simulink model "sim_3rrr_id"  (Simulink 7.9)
settings: Solver=ode45  StartTime=0.0  StopTime=2  RelTol=1e-3  AbsTol=1e-3
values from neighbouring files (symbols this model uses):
  m = 1    [mechanical_system.m]
  s = Lv/norm(Lv)    [pkm1.m]
undefined symbols (not defined in the file or in its folder): deg, kg, mN, N, rad
libraries: mblibv1 x26

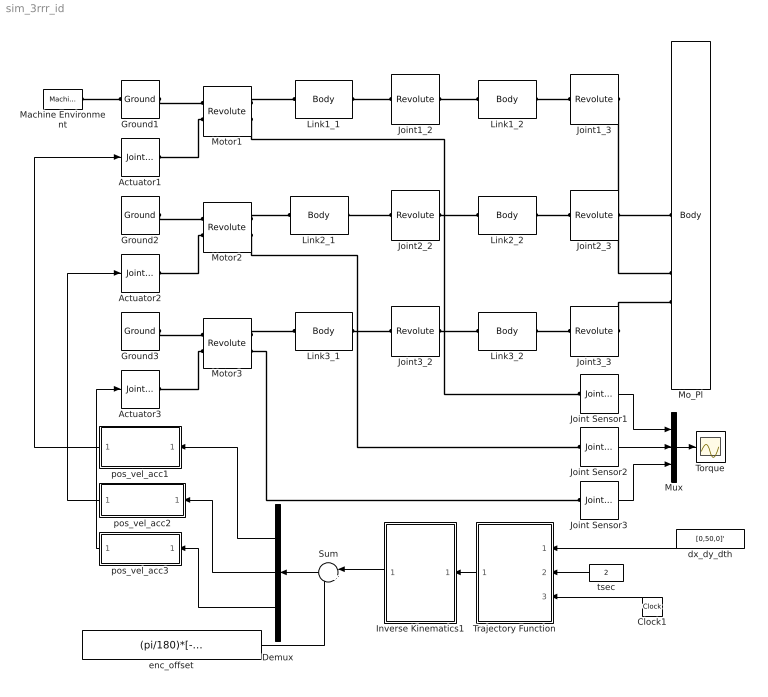
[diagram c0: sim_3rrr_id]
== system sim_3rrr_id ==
  Actuator1 : mblibv1/Sensors &  Actuators/Joint Actuator  UpdateFromCAD=off  PhysicalDomain=Mechanical  PortType=blob  ActuationStyle=Motion  AngleUnits=rad  ArcVelocityUnits=rad/s  ArcAccelerationUnits=rad/s^2  CoordPositionUnits=m  VelocityUnits=m/s  AccelerationUnits=m/s^2  ForceUnits=N  TorqueUnits=N*m  ActiveIO=on  Width=3  DialogClass=MechanicalActuatorBlock  Primitive=R1  ReferenceFrame=Absolute (World)
  Actuator2 : mblibv1/Sensors &  Actuators/Joint Actuator  UpdateFromCAD=off  PhysicalDomain=Mechanical  PortType=blob  ActuationStyle=Motion  AngleUnits=rad  ArcVelocityUnits=rad/s  ArcAccelerationUnits=rad/s^2  CoordPositionUnits=m  VelocityUnits=m/s  AccelerationUnits=m/s^2  ForceUnits=N  TorqueUnits=N*m  ActiveIO=on  Width=3  DialogClass=MechanicalActuatorBlock  Primitive=R1  ReferenceFrame=Absolute (World)
  Actuator3 : mblibv1/Sensors &  Actuators/Joint Actuator  UpdateFromCAD=off  PhysicalDomain=Mechanical  PortType=blob  ActuationStyle=Motion  AngleUnits=rad  ArcVelocityUnits=rad/s  ArcAccelerationUnits=rad/s^2  CoordPositionUnits=m  VelocityUnits=m/s  AccelerationUnits=m/s^2  ForceUnits=N  TorqueUnits=N*m  ActiveIO=on  Width=3  DialogClass=MechanicalActuatorBlock  Primitive=R1  ReferenceFrame=Absolute (World)
  Clock1 : Clock
  Demux : Demux  Outputs=3
  Ground1 : mblibv1/Bodies/Ground  UpdateFromCAD=off  LeftPortType=env  RightPortType=workingframe  PhysicalDomain=Mechanical  DialogClass=GroundBlock  CoordPosition=[0 0.15 0]  CoordPositionUnits=m  StateVectorMgrId=10  MachineId=[11 0]  ShowEnvPort=on
  Ground2 : mblibv1/Bodies/Ground  UpdateFromCAD=off  LeftPortType=env  RightPortType=workingframe  PhysicalDomain=Mechanical  DialogClass=GroundBlock  CoordPosition=[-0.1299 -0.075 0]  CoordPositionUnits=m  StateVectorMgrId=-1  MachineId=[0 0]  ShowEnvPort=off
  Ground3 : mblibv1/Bodies/Ground  UpdateFromCAD=off  LeftPortType=env  RightPortType=workingframe  PhysicalDomain=Mechanical  DialogClass=GroundBlock  CoordPosition=[0.129902 -0.074997 0]  CoordPositionUnits=m  StateVectorMgrId=-1  MachineId=[0 0]  ShowEnvPort=off
  Inverse Kinematics1 : MATLAB Function  TreatAsAtomicUnit=on
  Joint Sensor1 : mblibv1/Sensors &  Actuators/Joint Sensor  UpdateFromCAD=off  PhysicalDomain=Mechanical  PortType=blob  Muxed=on  Pose=off  Angle=off  AngleUnits=deg  ArcVelocity=off  ArcVelocityUnits=deg/s  ArcAcceleration=off  ArcAccelerationUnits=deg/s^2  CoordPosition=on  CoordPositionUnits=m  Velocity=off  VelocityUnits=m/s  Acceleration=off  AccelerationUnits=m/s^2  Quaternion=on  QuaternionDT=off  QuaternionDDT=off  QuaternionUnits=off  OutputVector=[1]  ActiveIO=on  Width=1  DialogClass=MechanicalSensorBlock  Primitive=R1  Force=off  ForceUnits=N  Torque=on  TorqueUnits=mN*m  ReferenceFrame=Absolute (World)  ReactionSensedSide=Base  ReactionReferenceFrame=Absolute (World)  ReactionForce=off  ReactionForceUnits=N  ReactionMoment=off  ReactionMomentUnits=N*m
  Joint Sensor2 : mblibv1/Sensors &  Actuators/Joint Sensor  UpdateFromCAD=off  PhysicalDomain=Mechanical  PortType=blob  Muxed=on  Pose=off  Angle=off  AngleUnits=deg  ArcVelocity=off  ArcVelocityUnits=deg/s  ArcAcceleration=off  ArcAccelerationUnits=deg/s^2  CoordPosition=on  CoordPositionUnits=m  Velocity=off  VelocityUnits=m/s  Acceleration=off  AccelerationUnits=m/s^2  Quaternion=on  QuaternionDT=off  QuaternionDDT=off  QuaternionUnits=off  OutputVector=[1]  ActiveIO=on  Width=1  DialogClass=MechanicalSensorBlock  Primitive=R1  Force=off  ForceUnits=N  Torque=on  TorqueUnits=mN*m  ReferenceFrame=Absolute (World)  ReactionSensedSide=Base  ReactionReferenceFrame=Absolute (World)  ReactionForce=off  ReactionForceUnits=N  ReactionMoment=off  ReactionMomentUnits=N*m
  Joint Sensor3 : mblibv1/Sensors &  Actuators/Joint Sensor  UpdateFromCAD=off  PhysicalDomain=Mechanical  PortType=blob  Muxed=on  Pose=off  Angle=off  AngleUnits=deg  ArcVelocity=off  ArcVelocityUnits=deg/s  ArcAcceleration=off  ArcAccelerationUnits=deg/s^2  CoordPosition=on  CoordPositionUnits=m  Velocity=off  VelocityUnits=m/s  Acceleration=off  AccelerationUnits=m/s^2  Quaternion=on  QuaternionDT=off  QuaternionDDT=off  QuaternionUnits=off  OutputVector=[1]  ActiveIO=on  Width=1  DialogClass=MechanicalSensorBlock  Primitive=R1  Force=off  ForceUnits=N  Torque=on  TorqueUnits=mN*m  ReferenceFrame=Absolute (World)  ReactionSensedSide=Base  ReactionReferenceFrame=Absolute (World)  ReactionForce=off  ReactionForceUnits=N  ReactionMoment=off  ReactionMomentUnits=N*m
  Joint1_2 : mblibv1/Joints/Revolute  LConnTagsString=__newl0  RConnTagsString=__newr0  UpdateFromCAD=off  NumSAPorts=0  CutJoint=off  MarkAsCut=off  Primitives=prismatic  PrimitiveProps=R1$World$[0 0 1]$revolute  DialogClass=JointBlock  R1Axis=[0 0 1]
  Joint1_3 : mblibv1/Joints/Revolute  LConnTagsString=__newl0  RConnTagsString=__newr0  UpdateFromCAD=off  NumSAPorts=0  CutJoint=off  MarkAsCut=off  Primitives=prismatic  PrimitiveProps=R1$World$[0 0 1]$revolute  DialogClass=JointBlock  R1Axis=[0 0 1]
  Joint2_2 : mblibv1/Joints/Revolute  LConnTagsString=__newl0  RConnTagsString=__newr0  UpdateFromCAD=off  NumSAPorts=0  CutJoint=off  MarkAsCut=off  Primitives=prismatic  PrimitiveProps=R1$World$[0 0 1]$revolute  DialogClass=JointBlock  R1Axis=[0 0 1]
  Joint2_3 : mblibv1/Joints/Revolute  LConnTagsString=__newl0  RConnTagsString=__newr0  UpdateFromCAD=off  NumSAPorts=0  CutJoint=off  MarkAsCut=off  Primitives=prismatic  PrimitiveProps=R1$World$[0 0 1]$revolute  DialogClass=JointBlock  R1Axis=[0 0 1]
  Joint3_2 : mblibv1/Joints/Revolute  LConnTagsString=__newl0  RConnTagsString=__newr0  UpdateFromCAD=off  NumSAPorts=0  CutJoint=off  MarkAsCut=off  Primitives=prismatic  PrimitiveProps=R1$World$[0 0 1]$revolute  DialogClass=JointBlock  R1Axis=[0 0 1]
  Joint3_3 : mblibv1/Joints/Revolute  LConnTagsString=__newl0  RConnTagsString=__newr0  UpdateFromCAD=off  NumSAPorts=0  CutJoint=off  MarkAsCut=off  Primitives=prismatic  PrimitiveProps=R1$World$[0 0 1]$revolute  DialogClass=JointBlock  R1Axis=[0 0 1]
  Link1_1 : mblibv1/Bodies/Body  LConnTagsString=CS1  RConnTagsString=CS2  UpdateFromCAD=off  DialogClass=MechanicalBodyBlock  Mass=0.053  MassUnits=kg  InertiaUnits=kg*m^2  Inertia=[0 0 0; 0 0 0; 0 0 0.000110621]  Shape=Cylinder  ShapeDims=[1 1]  ShapeUnits=m  ShapeUse=false  Density=1  DensityUnits=kg/m^3  DensityUse=false  GraphicsMode=MACHINE_DEFAULT  BodyColorSelMode=MACHINE_DEFAULT  BodyColor=[1 0 0]  AttachedToCS=CG  CG=Left$CG$[-0.043452 -0.030538 0]$CS1$CS1$m$[0 0 0]$Euler X-Y-Z$deg$WORLD$false$none  WorkingFrames=Left$CS1$[0 0.15 0]$World$World$m$[0 0 0]$Euler X-Y-Z$deg$WORLD$true$none#Right$CS2$[-0.081818 0.092497 0]$World$World$m$[0 0 0]$Euler X-Y-Z$deg$WORLD$true$none  CGPos=[-0.043452 -0.030538 0]  CGRot=[0 0 0]  CS0Pos=[]  CS0Rot=[]  CS1Pos=[0 0.15 0]  CS1Rot=[0 0 0]  CS2Pos=[-0.081818 0.092497 0]  CS2Rot=[0 0 0]  CS3Pos=[]  CS3Rot=[]  CS4Pos=[]  CS4Rot=[]  CS5Pos=[]  CS5Rot=[]  CS6Pos=[]  CS6Rot=[]  CS7Pos=[]  CS7Rot=[]  CS8Pos=[]  CS8Rot=[]  CS9Pos=[]  CS9Rot=[]  CS10Pos=[]  CS10Rot=[]  CS11Pos=[]  CS11Rot=[]  CS12Pos=[]  CS12Rot=[]  CS13Pos=[]  CS13Rot=[]  CS14Pos=[]  CS14Rot=[]  CS15Pos=[]  CS15Rot=[]  CS16Pos=[]  CS16Rot=[]  CS17Pos=[]  CS17Rot=[]  CS18Pos=[]  CS18Rot=[]  CS19Pos=[]  CS19Rot=[]  CS20Pos=[]  CS20Rot=[]
  Link1_2 : mblibv1/Bodies/Body  LConnTagsString=CS1  RConnTagsString=CS2  UpdateFromCAD=off  DialogClass=MechanicalBodyBlock  Mass=0.045  MassUnits=kg  InertiaUnits=kg*m^2  Inertia=[0 0 0; 0 0 0; 0 0 0.000090992]  Shape=Cylinder  ShapeDims=[1 1]  ShapeUnits=m  ShapeUse=false  Density=1  DensityUnits=kg/m^3  DensityUse=false  GraphicsMode=MACHINE_DEFAULT  BodyColorSelMode=MACHINE_DEFAULT  BodyColor=[1 0 0]  AttachedToCS=CG  CG=Left$CG$[0.040909 -0.028749 0]$CS1$CS1$m$[0 0 0]$Euler X-Y-Z$deg$WORLD$false$none  WorkingFrames=Left$CS1$[-0.081818 0.092497 0]$World$World$m$[0 0 0]$Euler X-Y-Z$deg$WORLD$true$none#Right$CS2$[0 0.035 0]$World$World$m$[0 0 0]$Euler X-Y-Z$deg$WORLD$true$none  CGPos=[0.040909 -0.028749 0]  CGRot=[0 0 0]  CS0Pos=[]  CS0Rot=[]  CS1Pos=[-0.081818 0.092497 0]  CS1Rot=[0 0 0]  CS2Pos=[0 0.035 0]  CS2Rot=[0 0 0]  CS3Pos=[]  CS3Rot=[]  CS4Pos=[]  CS4Rot=[]  CS5Pos=[]  CS5Rot=[]  CS6Pos=[]  CS6Rot=[]  CS7Pos=[]  CS7Rot=[]  CS8Pos=[]  CS8Rot=[]  CS9Pos=[]  CS9Rot=[]  CS10Pos=[]  CS10Rot=[]  CS11Pos=[]  CS11Rot=[]  CS12Pos=[]  CS12Rot=[]  CS13Pos=[]  CS13Rot=[]  CS14Pos=[]  CS14Rot=[]  CS15Pos=[]  CS15Rot=[]  CS16Pos=[]  CS16Rot=[]  CS17Pos=[]  CS17Rot=[]  CS18Pos=[]  CS18Rot=[]  CS19Pos=[]  CS19Rot=[]  CS20Pos=[]  CS20Rot=[]
  Link2_1 : mblibv1/Bodies/Body  LConnTagsString=CS1  RConnTagsString=CS2  UpdateFromCAD=off  DialogClass=MechanicalBodyBlock  Mass=0.053  MassUnits=kg  InertiaUnits=kg*m^2  Inertia=[0 0 0; 0 0 0; 0 0 0.000110621]  Shape=Cylinder  ShapeDims=[1 1]  ShapeUnits=m  ShapeUse=false  Density=1  DensityUnits=kg/m^3  DensityUse=false  GraphicsMode=MACHINE_DEFAULT  BodyColorSelMode=MACHINE_DEFAULT  BodyColor=[1 0 0]  AttachedToCS=CG  CG=Left$CG$[0.048173 -0.022361 0]$CS1$CS1$m$[0 0 0]$Euler X-Y-Z$deg$WORLD$false$none  WorkingFrames=Left$CS1$[-0.1299 -0.075 0]$World$World$m$[0 0 0]$Euler X-Y-Z$deg$WORLD$true$none#Right$CS2$[-0.039196 -0.117104 0]$World$World$m$[0 0 0]$Euler X-Y-Z$deg$WORLD$true$none  CGPos=[0.048173 -0.022361 0]  CGRot=[0 0 0]  CS0Pos=[]  CS0Rot=[]  CS1Pos=[-0.1299 -0.075 0]  CS1Rot=[0 0 0]  CS2Pos=[-0.039196 -0.117104 0]  CS2Rot=[0 0 0]  CS3Pos=[]  CS3Rot=[]  CS4Pos=[]  CS4Rot=[]  CS5Pos=[]  CS5Rot=[]  CS6Pos=[]  CS6Rot=[]  CS7Pos=[]  CS7Rot=[]  CS8Pos=[]  CS8Rot=[]  CS9Pos=[]  CS9Rot=[]  CS10Pos=[]  CS10Rot=[]  CS11Pos=[]  CS11Rot=[]  CS12Pos=[]  CS12Rot=[]  CS13Pos=[]  CS13Rot=[]  CS14Pos=[]  CS14Rot=[]  CS15Pos=[]  CS15Rot=[]  CS16Pos=[]  CS16Rot=[]  CS17Pos=[]  CS17Rot=[]  CS18Pos=[]  CS18Rot=[]  CS19Pos=[]  CS19Rot=[]  CS20Pos=[]  CS20Rot=[]
  Link2_2 : mblibv1/Bodies/Body  LConnTagsString=CS1  RConnTagsString=CS2  UpdateFromCAD=off  DialogClass=MechanicalBodyBlock  Mass=0.045  MassUnits=kg  InertiaUnits=kg*m^2  Inertia=[0 0 0; 0 0 0; 0 0 0.000090992]  Shape=Cylinder  ShapeDims=[1 1]  ShapeUnits=m  ShapeUse=false  Density=1  DensityUnits=kg/m^3  DensityUse=false  GraphicsMode=MACHINE_DEFAULT  BodyColorSelMode=MACHINE_DEFAULT  BodyColor=[1 0 0]  AttachedToCS=CG  CG=Left$CG$[0.0044425 0.049802 0]$CS1$CS1$m$[0 0 0]$Euler X-Y-Z$deg$WORLD$false$none  WorkingFrames=Left$CS1$[-0.039196 -0.117104 0]$World$World$m$[0 0 0]$Euler X-Y-Z$deg$WORLD$true$none#Right$CS2$[-0.03011 -0.0175 0]$World$World$m$[0 0 0]$Euler X-Y-Z$deg$WORLD$true$none  CGPos=[0.0044425 0.049802 0]  CGRot=[0 0 0]  CS0Pos=[]  CS0Rot=[]  CS1Pos=[-0.039196 -0.117104 0]  CS1Rot=[0 0 0]  CS2Pos=[-0.03011 -0.0175 0]  CS2Rot=[0 0 0]  CS3Pos=[]  CS3Rot=[]  CS4Pos=[]  CS4Rot=[]  CS5Pos=[]  CS5Rot=[]  CS6Pos=[]  CS6Rot=[]  CS7Pos=[]  CS7Rot=[]  CS8Pos=[]  CS8Rot=[]  CS9Pos=[]  CS9Rot=[]  CS10Pos=[]  CS10Rot=[]  CS11Pos=[]  CS11Rot=[]  CS12Pos=[]  CS12Rot=[]  CS13Pos=[]  CS13Rot=[]  CS14Pos=[]  CS14Rot=[]  CS15Pos=[]  CS15Rot=[]  CS16Pos=[]  CS16Rot=[]  CS17Pos=[]  CS17Rot=[]  CS18Pos=[]  CS18Rot=[]  CS19Pos=[]  CS19Rot=[]  CS20Pos=[]  CS20Rot=[]
  Link3_1 : mblibv1/Bodies/Body  LConnTagsString=CS1  RConnTagsString=CS2  UpdateFromCAD=off  DialogClass=MechanicalBodyBlock  Mass=0.053  MassUnits=kg  InertiaUnits=kg*m^2  Inertia=[0 0 0; 0 0 0; 0 0 0.000110621]  Shape=Cylinder  ShapeDims=[1 1]  ShapeUnits=m  ShapeUse=false  Density=1  DensityUnits=kg/m^3  DensityUse=false  GraphicsMode=MACHINE_DEFAULT  BodyColorSelMode=MACHINE_DEFAULT  BodyColor=[1 0 0]  AttachedToCS=CG  CG=Left$CG$[-0.0047204 0.0528997 0]$CS1$CS1$m$[0 0 0]$Euler X-Y-Z$deg$WORLD$false$none  WorkingFrames=Left$CS1$[0.129902 -0.074997 0]$World$World$m$[0 0 0]$Euler X-Y-Z$deg$WORLD$true$none#Right$CS2$[0.121013 0.024607 0]$World$World$m$[0 0 0]$Euler X-Y-Z$deg$WORLD$true$none  CGPos=[-0.0047204 0.0528997 0]  CGRot=[0 0 0]  CS0Pos=[]  CS0Rot=[]  CS1Pos=[0.129902 -0.074997 0]  CS1Rot=[0 0 0]  CS2Pos=[0.121013 0.024607 0]  CS2Rot=[0 0 0]  CS3Pos=[]  CS3Rot=[]  CS4Pos=[]  CS4Rot=[]  CS5Pos=[]  CS5Rot=[]  CS6Pos=[]  CS6Rot=[]  CS7Pos=[]  CS7Rot=[]  CS8Pos=[]  CS8Rot=[]  CS9Pos=[]  CS9Rot=[]  CS10Pos=[]  CS10Rot=[]  CS11Pos=[]  CS11Rot=[]  CS12Pos=[]  CS12Rot=[]  CS13Pos=[]  CS13Rot=[]  CS14Pos=[]  CS14Rot=[]  CS15Pos=[]  CS15Rot=[]  CS16Pos=[]  CS16Rot=[]  CS17Pos=[]  CS17Rot=[]  CS18Pos=[]  CS18Rot=[]  CS19Pos=[]  CS19Rot=[]  CS20Pos=[]  CS20Rot=[]
  Link3_2 : mblibv1/Bodies/Body  LConnTagsString=CS1  RConnTagsString=CS2  UpdateFromCAD=off  DialogClass=MechanicalBodyBlock  Mass=0.045  MassUnits=kg  InertiaUnits=kg*m^2  Inertia=[0 0 0; 0 0 0; 0 0 0.000090992]  Shape=Cylinder  ShapeDims=[1 1]  ShapeUnits=m  ShapeUse=false  Density=1  DensityUnits=kg/m^3  DensityUse=false  GraphicsMode=MACHINE_DEFAULT  BodyColorSelMode=MACHINE_DEFAULT  BodyColor=[1 0 0]  AttachedToCS=CG  CG=Left$CG$[-0.0453515 -0.0210535 0]$CS1$CS1$m$[0 0 0]$Euler X-Y-Z$deg$WORLD$false$none  WorkingFrames=Left$CS1$[0.121013 0.024607 0]$World$World$m$[0 0 0]$Euler X-Y-Z$deg$WORLD$true$none#Right$CS2$[0.030311 -0.0175 0]$World$World$m$[0 0 0]$Euler X-Y-Z$deg$WORLD$true$none  CGPos=[-0.0453515 -0.0210535 0]  CGRot=[0 0 0]  CS0Pos=[]  CS0Rot=[]  CS1Pos=[0.121013 0.024607 0]  CS1Rot=[0 0 0]  CS2Pos=[0.030311 -0.0175 0]  CS2Rot=[0 0 0]  CS3Pos=[]  CS3Rot=[]  CS4Pos=[]  CS4Rot=[]  CS5Pos=[]  CS5Rot=[]  CS6Pos=[]  CS6Rot=[]  CS7Pos=[]  CS7Rot=[]  CS8Pos=[]  CS8Rot=[]  CS9Pos=[]  CS9Rot=[]  CS10Pos=[]  CS10Rot=[]  CS11Pos=[]  CS11Rot=[]  CS12Pos=[]  CS12Rot=[]  CS13Pos=[]  CS13Rot=[]  CS14Pos=[]  CS14Rot=[]  CS15Pos=[]  CS15Rot=[]  CS16Pos=[]  CS16Rot=[]  CS17Pos=[]  CS17Rot=[]  CS18Pos=[]  CS18Rot=[]  CS19Pos=[]  CS19Rot=[]  CS20Pos=[]  CS20Rot=[]
  Machine Environment : mblibv1/Bodies/Machine Environment  PortType=env  PhysicalDomain=Mechanical  DialogTemplateClass=MECH.MachineEnvironment  SyncWhenCopied=off  Gravity=[0 -9.81 0]  GravityUnits=m/s^2  GravityAsSignal=off  Dimensionality=Auto-detect  AnalysisType=Forward dynamics  LinearAssemblyTolerance=1e-3  LinearAssemblyToleranceUnits=m  AngularAssemblyTolerance=1e-3  AngularAssemblyToleranceUnits=rad  ConstraintSolverType=Stabilizing  ConstraintRelTolerance=1e-4  ConstraintAbsTolerance=1e-4  UseRobustSingularityHandling=off  RedundancyAnalysisToleranceType=Automatically select tolerance  RedundancyAnalysisTolerance=1e-14  StatePerturbationType=Fixed  PerturbationSize=1e-5  VisualizeMachine=on  BodyVisualizationType=Use model default body geometries  BodyColorSelMode=Use model default  DefaultBodyColor=[1 0 0]
  Mo_Pl : mblibv1/Bodies/Body  LConnTagsString=CS1|CS2|CS3  UpdateFromCAD=off  DialogClass=MechanicalBodyBlock  Mass=0.081  MassUnits=kg  InertiaUnits=kg*m^2  Inertia=[0.000046643 0 0; 0 0.000046643 0; 0 0 0]  Shape=Cylinder  ShapeDims=[1 1]  ShapeUnits=m  ShapeUse=false  Density=1  DensityUnits=kg/m^3  DensityUse=false  GraphicsMode=MACHINE_DEFAULT  BodyColorSelMode=MACHINE_DEFAULT  BodyColor=[1 0 0]  AttachedToCS=CG  CG=Left$CG$[0 0 0]$WORLD$WORLD$m$[0 0 0]$Euler X-Y-Z$deg$WORLD$false$none  WorkingFrames=Left$CS1$[0 0.035 0]$World$World$m$[0 0 0]$Euler X-Y-Z$deg$WORLD$true$none#Left$CS2$[-0.03011 -0.0175 0]$World$World$m$[0 0 0]$Euler X-Y-Z$deg$WORLD$true$none#Left$CS3$[0.030311 -0.0175 0]$World$World$m$[0 0 0]$Euler X-Y-Z$deg$WORLD$true$none  CGPos=[0 0 0]  CGRot=[0 0 0]  CS0Pos=[]  CS0Rot=[]  CS1Pos=[0 0.035 0]  CS1Rot=[0 0 0]  CS2Pos=[-0.03011 -0.0175 0]  CS2Rot=[0 0 0]  CS3Pos=[0.030311 -0.0175 0]  CS3Rot=[0 0 0]  CS4Pos=[]  CS4Rot=[]  CS5Pos=[]  CS5Rot=[]  CS6Pos=[]  CS6Rot=[]  CS7Pos=[]  CS7Rot=[]  CS8Pos=[]  CS8Rot=[]  CS9Pos=[]  CS9Rot=[]  CS10Pos=[]  CS10Rot=[]  CS11Pos=[]  CS11Rot=[]  CS12Pos=[]  CS12Rot=[]  CS13Pos=[]  CS13Rot=[]  CS14Pos=[]  CS14Rot=[]  CS15Pos=[]  CS15Rot=[]  CS16Pos=[]  CS16Rot=[]  CS17Pos=[]  CS17Rot=[]  CS18Pos=[]  CS18Rot=[]  CS19Pos=[]  CS19Rot=[]  CS20Pos=[]  CS20Rot=[]
  Motor1 : mblibv1/Joints/Revolute  LConnTagsString=__newl0|SA1  RConnTagsString=__newr0|SA1  UpdateFromCAD=off  NumSAPorts=2  CutJoint=off  MarkAsCut=off  Primitives=prismatic  PrimitiveProps=R1$World$[0 0 1]$revolute  DialogClass=JointBlock  R1Axis=[0 0 1]
  Motor2 : mblibv1/Joints/Revolute  LConnTagsString=__newl0|SA1  RConnTagsString=__newr0|SA1  UpdateFromCAD=off  NumSAPorts=2  CutJoint=off  MarkAsCut=off  Primitives=prismatic  PrimitiveProps=R1$World$[0 0 1]$revolute  DialogClass=JointBlock  R1Axis=[0 0 1]
  Motor3 : mblibv1/Joints/Revolute  LConnTagsString=__newl0|SA1  RConnTagsString=__newr0|SA1  UpdateFromCAD=off  NumSAPorts=2  CutJoint=off  MarkAsCut=off  Primitives=prismatic  PrimitiveProps=R1$World$[0 0 1]$revolute  DialogClass=JointBlock  R1Axis=[0 0 1]
  Mux : Mux  Inputs=3
  Sum : Sum  Inputs=|+-
  Torque : Scope
  Trajectory Function : MATLAB Function  TreatAsAtomicUnit=on
  dx_dy_dth : Constant  Value=[0,50,0]'  SampleTime=-1
  enc_offset : Constant  Value=(pi/180)*[-144.9004,-24.9004,95.0996]'
  pos_vel_acc1 : Subsystem
  pos_vel_acc2 : Subsystem
  pos_vel_acc3 : Subsystem
  tsec : Constant  Value=2  SampleTime=-1
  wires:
  Joint Sensor2/1 -> Mux/2
  pos_vel_acc1/1(Motion1) -> Actuator1/1
  pos_vel_acc2/1(Motion2) -> Actuator2/1
  pos_vel_acc3/1(Motion3) -> Actuator3/1
  Demux/1 -> pos_vel_acc1/1(In1)
  Demux/2 -> pos_vel_acc2/1(In1)
  Demux/3 -> pos_vel_acc3/1(In1)
  Sum/1 -> Demux/1
  Inverse Kinematics1/1(thd) -> Sum/1
  Trajectory Function/1(xd) -> Inverse Kinematics1/1(xd)
  dx_dy_dth/1 -> Trajectory Function/1(dx)
  tsec/1 -> Trajectory Function/2(tsec)
  Clock1/1 -> Trajectory Function/3(tout)
  enc_offset/1 -> Sum/2
  Mux/1 -> Torque/1
  Joint Sensor1/1 -> Mux/1
  Joint Sensor3/1 -> Mux/3
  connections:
  Machine Environment/RConn1 -- Ground1/LConn1
  Ground1/RConn1 -- Motor1/LConn1
  Motor1/RConn1 -- Link1_1/LConn1
  Link1_1/RConn1 -- Joint1_2/LConn1
  Joint1_2/RConn1 -- Link1_2/LConn1
  Joint1_3/RConn1 -- Mo_Pl/LConn1
  Link1_2/RConn1 -- Joint1_3/LConn1
  Motor2/RConn1 -- Link2_1/LConn1
  Ground2/RConn1 -- Motor2/LConn1
  Link2_2/RConn1 -- Joint2_3/LConn1
  Joint2_2/RConn1 -- Link2_2/LConn1
  Link2_1/RConn1 -- Joint2_2/LConn1
  Joint2_3/RConn1 -- Mo_Pl/LConn2
  Link3_1/RConn1 -- Joint3_2/LConn1
  Motor3/RConn1 -- Link3_1/LConn1
  Ground3/RConn1 -- Motor3/LConn1
  Joint3_2/RConn1 -- Link3_2/LConn1
  Link3_2/RConn1 -- Joint3_3/LConn1
  Joint3_3/RConn1 -- Mo_Pl/LConn3
  Motor1/RConn2 -- Joint Sensor1/LConn1
  Motor2/RConn2 -- Joint Sensor2/LConn1
  Motor3/RConn2 -- Joint Sensor3/LConn1
  Motor1/LConn2 -- Actuator1/RConn1
  Motor2/LConn2 -- Actuator2/RConn1
  Motor3/LConn2 -- Actuator3/RConn1

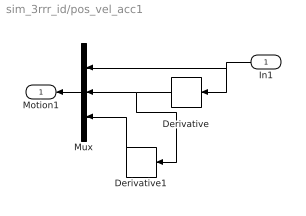
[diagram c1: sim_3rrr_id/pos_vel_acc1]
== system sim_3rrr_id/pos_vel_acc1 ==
  In1 : Inport
  Derivative : Derivative
  Derivative1 : Derivative
  Mux : Mux  Inputs=3
  Motion1 : Outport
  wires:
  Mux/1 -> Motion1/1
  Derivative/1 -> Mux/2, Derivative1/1
  Derivative1/1 -> Mux/3
  In1/1 -> Mux/1, Derivative/1

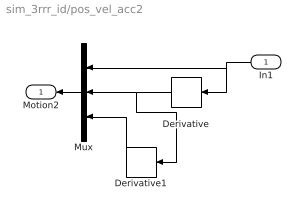
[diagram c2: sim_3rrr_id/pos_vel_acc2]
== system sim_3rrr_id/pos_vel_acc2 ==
  In1 : Inport
  Derivative : Derivative
  Derivative1 : Derivative
  Mux : Mux  Inputs=3
  Motion2 : Outport
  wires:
  Mux/1 -> Motion2/1
  Derivative/1 -> Mux/2, Derivative1/1
  Derivative1/1 -> Mux/3
  In1/1 -> Mux/1, Derivative/1

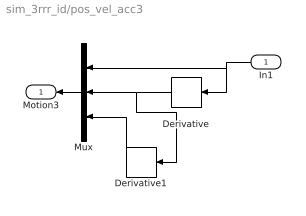
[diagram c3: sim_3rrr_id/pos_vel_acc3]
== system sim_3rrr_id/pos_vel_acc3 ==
  In1 : Inport
  Derivative : Derivative
  Derivative1 : Derivative
  Mux : Mux  Inputs=3
  Motion3 : Outport
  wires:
  Mux/1 -> Motion3/1
  Derivative/1 -> Mux/2, Derivative1/1
  Derivative1/1 -> Mux/3
  In1/1 -> Mux/1, Derivative/1

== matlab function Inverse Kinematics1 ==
function thd = fcn(xd)

persistent index thd_p

% Initializing Variables %
if isempty(index), index=0; end
if isempty(thd_p), thd_p=(pi/180)*[-144.9004,-24.9004,95.0996]'; end

% Kinematic Parameters %
ra=150; rb=35; L1=100; L2=100;

pos=xd(1:2,1); ang=xd(3,1);

w_index=1;  % In workspace %

% Vertex Points %
A=ra*[0,-sqrt(3)/2, +sqrt(3)/2; 1, -1/2, -1/2];
B=rb*[0,-sqrt(3)/2, +sqrt(3)/2; 1, -1/2, -1/2];

th=zeros(3,1);
R=[cos(ang), -sin(ang); sin(ang), cos(ang)];
for i=1:3
    d=pos+R*B(:,i)-A(:,i);
    e1=-2*L1*d(2,1); e2=-2*L1*d(1,1);
    e3=d(1,1)^2+d(2,1)^2+L1^2-L2^2;
    temp=e1^2+e2^2-e3^2;
    if temp>=0
        th(i,1)=2*atan((-e1-sqrt(temp))/(e3-e2));
    else
        th(i,1)=0;
        w_index=-1;
        %disp('Out of Workspace');
    end
end

% Result %
if w_index==1
    thd=[th(1,1), th(2,1), th(3,1)]';
else
    thd=thd_p;
end

% Save the current value %
thd_p=thd;

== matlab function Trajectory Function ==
function xd = fcn(dx, tsec, tout)

MAX_CH=3;       % Two Actuators %


% Initializing Variables %
xd=zeros(MAX_CH,1);
x0=[0,0,0]';

%tout=index*dt;

    [c] = coeff_3rd(x0, zeros(MAX_CH,1), x0+dx, zeros(MAX_CH,1), tsec);
    for ch=1:MAX_CH
        xd(ch,1)=c(ch,1)+c(ch,2)*tout+c(ch,3)*tout^2+c(ch,4)*tout^3;    
    end

function [c] = coeff_3rd(sp, sv, ep, ev, tsec)
MAX_CH=3;
c=zeros(MAX_CH,4);
for ch=1:MAX_CH
    c(ch,1)=sp(ch,1);
    c(ch,2)=sv(ch,1);
    c(ch,3)=(3.0*(ep(ch,1)-sp(ch,1))-(2.0*sv(ch,1)+ev(ch,1))*tsec)/(tsec*tsec);
    c(ch,4)=(-2.0*(ep(ch,1)-sp(ch,1))+(sv(ch,1)+ev(ch,1))*tsec)/(tsec*tsec*tsec);
end
